PROGRAM PRG_READ
VAR
	(* Declarations for UA_Connect *)
	fbUA_Connect			: UA_Connect;
	SessionConnectInfo		: ST_UASessionConnectInfo;
	nConnectionHdl			: DWORD;

	(* Declarations for UA_GetNamespaceIndex *)
	fbUA_GetNamespaceIndex 	: UA_GetNamespaceIndex;
	nNamespaceIndex			: UINT;

	(* Declarations for UA_NodeGetHandle *)
	fbUA_NodeGetHandle		: UA_NodeGetHandle;
	NodeID					: ST_UANodeID;
	nNodeHdl				: DWORD;

	(* Declarations for UA_Read *)
	fbUA_Read				: UA_Read;
	stIndexRange			: ARRAY [1..nMaxIndexRange] OF ST_UAIndexRange;
	nIndexRangeCount		: UINT;
	stNodeAddInfo			: ST_UANodeAdditionalInfo;
	sNodeIdentifier			: STRING(MAX_STRING_LENGTH) := 'MAIN.nCounter'; // change to node identifier
	nReadData				: INT; 		// change to node data type
	cbDataRead				: UDINT;
	
	(* Declarations for UA_NodeReleaseHandle *)
	fbUA_NodeReleaseHandle	: UA_NodeReleaseHandle;

	(* Declarations for UA_Disconnect *)
	fbUA_Disconnect		: UA_Disconnect;

	(* Other declarations *)
	iState		: INT;
	bTest		: BOOL:= TRUE;
	bDone		: BOOL;
	bBusy		: BOOL;
	bError		: BOOL;
	nErrorID	: DWORD;
END_VAR


CASE iState OF
0:	(* idle *)
	IF bTest THEN
		bTest		:= FALSE;
		bError		:= FALSE;
		nErrorID	:= 0;

		SessionConnectInfo.tConnectTimeout 		:= T#1M;
		SessionConnectInfo.tSessionTimeout 		:= T#1M;
		SessionConnectInfo.sApplicationName		:= '';
		SessionConnectInfo.eSecurityMode 		:= eUASecurityMsgMode_None;
		SessionConnectInfo.eSecurityPolicyUri 	:= eUASecurityPolicy_None;
		SessionConnectInfo.eTransportProfileUri := eUATransportProfileUri_UATcp;

(*		nIndexRange[1].nStartIndex := 0;
		nIndexRange[1].nEndIndex := 1;
		nIndexRange[1].bRangeAccess := TRUE; *)
		stNodeAddInfo.nIndexRangeCount := nIndexRangeCount;
		stNodeAddInfo.stIndexRange := stIndexRange;
		iState	:= iState + 1;
	END_IF

1:	(* Open UA session *)
	fbUA_Connect(
		Execute				:= TRUE,
		ServerURL			:= sOpcUaServerUrl,
		SessionConnectInfo	:= SessionConnectInfo,
		Timeout				:= T#2M,
		ConnectionHdl		=> nConnectionHdl
	);

	IF NOT fbUA_Connect.Busy THEN
		fbUA_Connect(Execute := FALSE);

		IF NOT fbUA_Connect.Error THEN
			(* session open *)
			iState := iState + 1;
		ELSE
			bError			:= TRUE;
			nErrorID		:= fbUA_Connect.ErrorID;
			nConnectionHdl	:= 0;
			iState 			:= 0; (* idle *)
		END_IF
	END_IF


2:	(* GetNS Index *)
	fbUA_GetNamespaceIndex(
		Execute			:= TRUE,
		ConnectionHdl	:= nConnectionHdl,
		NamespaceUri	:= sNamespaceUri,
		NamespaceIndex	=> nNamespaceIndex
	);

	IF NOT fbUA_GetNamespaceIndex.Busy THEN
		fbUA_GetNamespaceIndex(Execute := FALSE);
		IF NOT fbUA_GetNamespaceIndex.Error THEN
			iState 		:= iState + 1;
		ELSE
			bError		:= TRUE;
			nErrorID	:= fbUA_GetNamespaceIndex.ErrorID;
			iState 		:= 6; (* idle *)
		END_IF
	END_IF

3:	(* Get Node Handle *)
	NodeID.eIdentifierType := eUAIdentifierType_String;
	NodeID.nNamespaceIndex := nNamespaceIndex;
	NodeID.sIdentifier	:= sNodeIdentifier;
	fbUA_NodeGetHandle(
		Execute			:= TRUE,
		ConnectionHdl	:= nConnectionHdl,
		NodeID			:= NodeID,
		NodeHdl			=> nNodeHdl
	);

	IF NOT fbUA_NodeGetHandle.Busy THEN
		fbUA_NodeGetHandle(Execute := FALSE);

		IF NOT fbUA_NodeGetHandle.Error THEN
			iState 		:= iState + 1;
		ELSE
			bError		:= TRUE;
			nErrorID	:= fbUA_NodeGetHandle.ErrorID;
			iState 		:= 6; (* idle *)
		END_IF
	END_IF


4: 	(* UA_Read *)
	fbUA_Read(
		Execute			:= TRUE,
		ConnectionHdl	:= nConnectionHdl,
		NodeHdl			:= nNodeHdl,
		cbData			:= SIZEOF(nReadData),
		stNodeAddInfo 	:= stNodeAddInfo,
		pVariable		:= ADR(nReadData)
		);

	IF NOT fbUA_Read.Busy THEN
		fbUA_Read( Execute := FALSE, cbData_R => cbDataRead);

		IF NOT fbUA_Read.Error THEN
			iState 		:= iState + 1;
		ELSE
			bError		:= TRUE;
			nErrorID	:= fbUA_Read.ErrorID;
			iState 		:= 6; (* idle *)
		END_IF
	END_IF


5:	(* Release Node Handle *)
	fbUA_NodeReleaseHandle(
		Execute			:= TRUE,
		ConnectionHdl	:= nConnectionHdl,
		NodeHdl			:= nNodeHdl
	);

	IF NOT fbUA_NodeReleaseHandle.Busy THEN
		fbUA_NodeReleaseHandle(Execute := FALSE);

		IF NOT fbUA_NodeReleaseHandle.Error THEN
			iState 		:= iState + 1;
		ELSE
			bError		:= TRUE;
			nErrorID	:= fbUA_NodeReleaseHandle.ErrorID;
			iState 		:= 6; (* idle *)
		END_IF
	END_IF


6:	(* close session *)
	fbUA_Disconnect(
		Execute			:= TRUE,
		ConnectionHdl	:= nConnectionHdl
	);

	IF NOT fbUA_Disconnect.Busy THEN
		fbUA_Disconnect(Execute := FALSE);
		bBusy := FALSE;
		IF NOT fbUA_Disconnect.Error THEN
			(* session closed *)
			iState 		:= 0;
			IF NOT bError THEN 
				bDone 	:= TRUE;
			END_IF
		ELSE
			bError			:= TRUE;
			nErrorID		:= fbUA_Disconnect.ErrorID;
			iState 			:= 0; (* idle *)
			nConnectionHdl	:= 0;
		END_IF
	END_IF
END_CASE

END_PROGRAM
